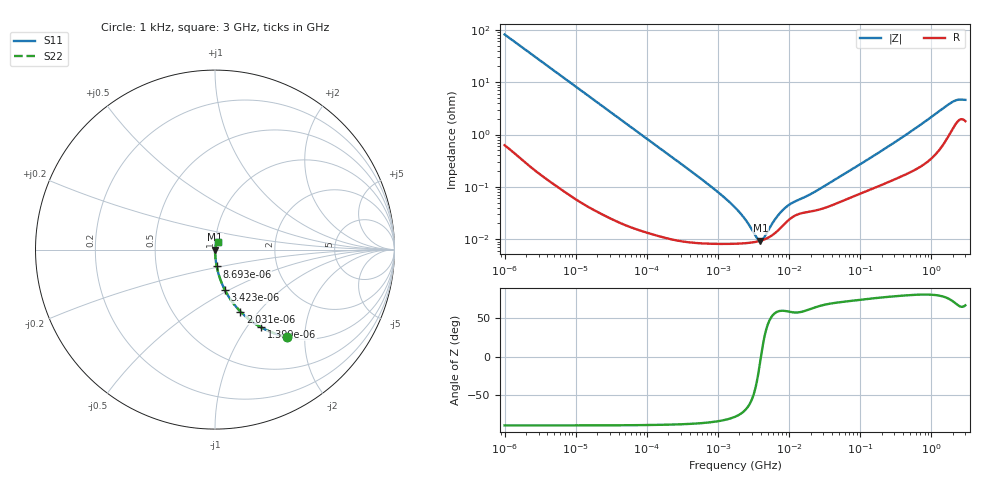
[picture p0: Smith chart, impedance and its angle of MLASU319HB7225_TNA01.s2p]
! MLASU319HB7225_TNA01  S-PARAMETER MODEL  ( Standard Model )
! Model Generated by TAIYO YUDEN Corporation (http://www.ty-top.com)
! Version 1.0
! TAIYO YUDEN Control No. 220601
! Copyright(c) 2011 TAIYO YUDEN CO.,LTD. All Rights Reserved.
! Product Description (link to TY-COMPAS)
! https://ds.yuden.co.jp/TYCOMPAS/or/detail?pn=MLASU319HB7225KTNA01&u=M
! Products Name : Multilayer Ceramic Capacitors
! Characteristics :
!  Capacitance : 2.2 [uF] , Rated Voltage : 50 [V] , TCC : X7R
!  Case Size : 3.2 x 1.6 / 0.126 x 0.063 [mm/inch] , Thickness : 0.85 / 0.033 [mm/inch]
!  (Conditions: Temperature = 25 [degC] , DC Bias Voltage = 0 [V])
! External Node Assignments :
!  1  o---| |---o  2
! GND o---------o GND
! Frequency Range : 1kHz  -  3GHz  [ 401 STEP ]
# MHZ S RI R 50
! Freq[MHz].  S11 Real  S11 Imag  S21 Real  S21 Imag  S12 Real  S12 Imag  S22 Real  S22 Imag
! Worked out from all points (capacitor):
!   401 points, 1 kHz to 3 GHz, reference 50 ohm
!   read as one part in series: C = 1.94 uF near 1.077 kHz
!   lowest |Z| = 9.36 mohm at 3.934 MHz (marker M1)
!   series resonance near 4.015 MHz, so ESL is about 810 pH
!   S11 on the Smith chart (normalised r, x): 1 kHz: 1.01, -1.63; 1.399 kHz: 1.01, -1.17; 2.031 kHz: 1.01, -0.81; 3.423 kHz: 1.00, -0.48; 8.693 kHz: 1.00, -0.19; 3 GHz: 1.04, +0.08
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0.001  0.4011 -0.4863  0.5989 0.4863  0.5989 0.4863  0.4011 -0.4863
0.001399  0.2567 -0.4332  0.7433 0.4332  0.7433 0.4332  0.2567 -0.4332
0.002031  0.1419 -0.3455  0.8581 0.3455  0.8581 0.3455  0.1419 -0.3455
0.003423  0.0558 -0.2263  0.9442 0.2263  0.9442 0.2263  0.0558 -0.2263
0.008693  0.00955 -0.0939  0.9904 0.0939  0.9904 0.0939  0.00955 -0.0939
0.01216  0.00507 -0.0675  0.9949 0.0675  0.9949 0.0675  0.00507 -0.0675
0.033275  0.000855 -0.0249  0.9991 0.0249  0.9991 0.0249  0.000855 -0.0249
0.147855  0.000146 -0.00563  0.9999 0.00563  0.9999 0.00563  0.000146 -0.00563
0.791611  8.28e-05 -0.00102  0.9999 0.00102  0.9999 0.00102  8.28e-05 -0.00102
1.732051  8.19e-05 -0.000396  0.9999 0.000396  0.9999 0.000396  8.19e-05 -0.000396
2.422679  8.38e-05 -0.000222  0.9999 0.000222  0.9999 0.000222  8.38e-05 -0.000222
3.388684  8.88e-05 -7.23e-05  0.9999 7.23e-05  0.9999 7.23e-05  8.88e-05 -7.23e-05
3.93371  9.32e-05 -8.69e-06  0.9999 8.69e-06  0.9999 8.69e-06  9.32e-05 -8.69e-06
4.566395  9.99e-05 5.52e-05  0.9999 -5.52e-05  0.9999 -5.52e-05  9.99e-05 5.52e-05
6.387174  0.000132 0.000204  0.9999 -0.000204  0.9999 -0.000204  0.000132 0.000204
8.606987  0.000195 0.000334  0.9998 -0.000334  0.9998 -0.000334  0.000195 0.000334
11.1738  0.000265 0.000422  0.9997 -0.000422  0.9997 -0.000422  0.000265 0.000422
21.06097  0.000343 0.000671  0.9997 -0.000671  0.9997 -0.000671  0.000343 0.000671
256.0921  0.00129 0.00595  0.9987 -0.00595  0.9987 -0.00595  0.00129 0.00595
1847.629  0.0121 0.0374  0.9879 -0.0374  0.9879 -0.0374  0.0121 0.0374
2310.849  0.0189 0.041  0.9811 -0.041  0.9811 -0.041  0.0189 0.041
3000  0.0194 0.0407  0.9806 -0.0407  0.9806 -0.0407  0.0194 0.0407
